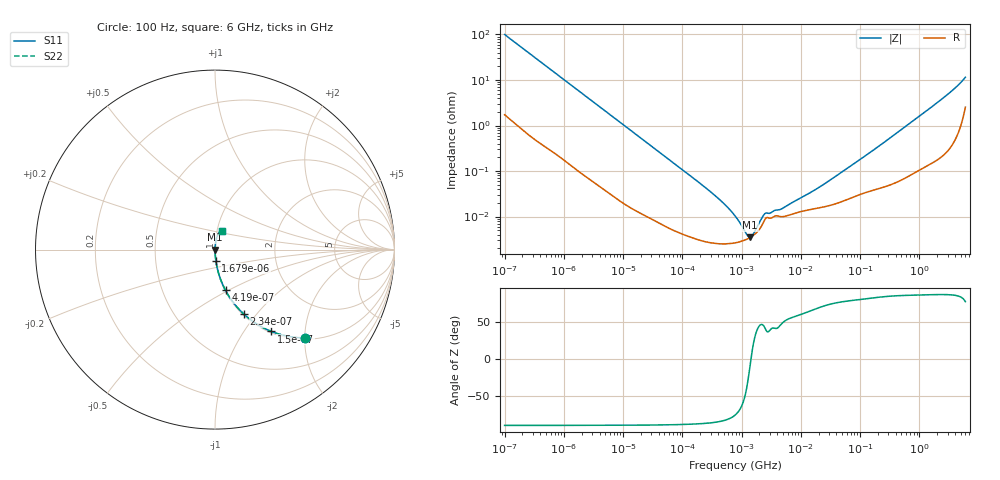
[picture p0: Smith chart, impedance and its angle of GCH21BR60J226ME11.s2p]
!Murata Part Number: GCH21BR60J226ME11
!These Parameters are Measured in Series Mode Connection
!Data Generated on Jun 19, 2026
!  o--ll--o
!Port1  Port2
!  o------o
!Operation Temp=25[degC], DC Bias Voltage=0[V]
!Freq. Start=100[Hz] Stop=6[GHz] 401[Steps]
# Hz S RI R 50
!Freq.(Hz) S11(Real) S11(Imag) S21(Real) S21(Imag) S12(Real) S12(Imag) S22(Real) S22(Imag)
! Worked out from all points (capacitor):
!   401 points, 100 Hz to 6 GHz, reference 50 ohm
!   read as one part in series: C = 15.8 uF near 109 Hz
!   lowest |Z| = 3.52 mohm at 1.386 MHz (marker M1)
!   series resonance near 1.44 MHz, so ESL is about 770 pH
!   S11 on the Smith chart (normalised r, x): 100 Hz: 1.03, -2.00; 150 Hz: 1.02, -1.34; 234 Hz: 1.01, -0.86; 419 Hz: 1.01, -0.48; 1.679 kHz: 1.00, -0.12; 6 GHz: 1.05, +0.22
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100  0.5007 -0.4915  0.4993 0.4915  0.4993 0.4915  0.5007 -0.4915
150  0.314 -0.4559  0.686 0.4559  0.686 0.4559  0.314 -0.4559
234  0.1607 -0.3595  0.8393 0.3595  0.8393 0.3595  0.1607 -0.3595
419  0.0586 -0.2271  0.9414 0.2271  0.9414 0.2271  0.0586 -0.2271
784  0.0188 -0.1275  0.9812 0.1275  0.9812 0.1275  0.0188 -0.1275
1679  0.00477 -0.061  0.9952 0.061  0.9952 0.061  0.00477 -0.061
2008  0.0035 -0.0512  0.9965 0.0512  0.9965 0.0512  0.0035 -0.0512
6433  0.000558 -0.0162  0.9994 0.0162  0.9994 0.0162  0.000558 -0.0162
40335  7.88e-05 -0.00264  0.9999 0.00264  0.9999 0.00264  7.88e-05 -0.00264
316350  2.64e-05 -0.000329  1 0.000329  1 0.000329  2.64e-05 -0.000329
495019  2.51e-05 -0.000195  1 0.000195  1 0.000195  2.51e-05 -0.000195
774597  2.64e-05 -0.000101  1 0.000101  1 0.000101  2.64e-05 -0.000101
885955  2.74e-05 -7.7e-05  1 7.7e-05  1 7.7e-05  2.74e-05 -7.7e-05
1386327  3.47e-05 -5.8e-06  1 5.8e-06  1 5.8e-06  3.47e-05 -5.8e-06
2074311  5.61e-05 5.83e-05  0.9999 -5.83e-05  0.9999 -5.83e-05  5.61e-05 5.83e-05
2594782  9.35e-05 7.52e-05  0.9999 -7.52e-05  0.9999 -7.52e-05  9.35e-05 7.52e-05
4643984  9.95e-05 0.000106  0.9999 -0.000106  0.9999 -0.000106  9.95e-05 0.000106
1.555665e7  0.000145 0.000324  0.9999 -0.000324  0.9999 -0.000324  0.000145 0.000324
3.80911e7  0.00019 0.000731  0.9998 -0.000731  0.9998 -0.000731  0.00019 0.000731
3.124326e8  0.000514 0.00517  0.9995 -0.00517  0.9995 -0.00517  0.000514 0.00517
2.34314e9  0.00339 0.037  0.9966 -0.037  0.9966 -0.037  0.00339 0.037
6e9  0.0363 0.1056  0.9637 -0.1056  0.9637 -0.1056  0.0363 0.1056
